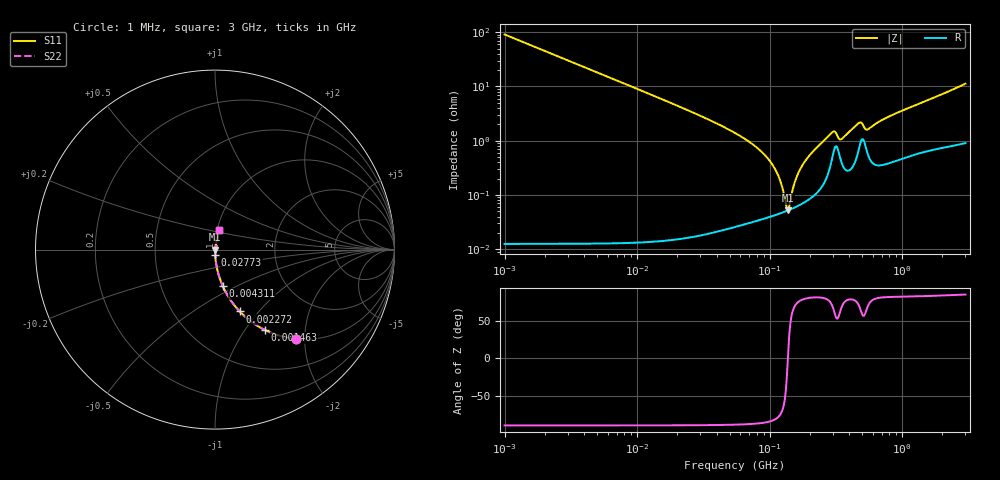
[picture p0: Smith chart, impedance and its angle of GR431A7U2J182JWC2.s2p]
!Murata Part Number: GR431A7U2J182JWC2
!These Parameters are Measured in Series Mode Connection
!Data Generated on Jun 10, 2025
!  o--ll--o
!Port1  Port2
!  o------o
!Operation Temp=25[degC], DC Bias Voltage=0[V]
!Freq. Start=1000[kHz] Stop=3[GHz] 401[Steps]
# Hz S RI R 50
!Freq.(Hz) S11(Real) S11(Imag) S21(Real) S21(Imag) S12(Real) S12(Imag) S22(Real) S22(Imag)
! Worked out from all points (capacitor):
!   401 points, 1 MHz to 3 GHz, reference 50 ohm
!   read as one part in series: C = 1.75 nF near 1.041 MHz
!   lowest |Z| = 52.1 mohm at 137.5 MHz (marker M1)
!   series resonance near 137.3 MHz, so ESL is about 770 pH
!   S11 on the Smith chart (normalised r, x): 1 MHz: 1.00, -1.82; 1.463 MHz: 1.00, -1.24; 2.272 MHz: 1.00, -0.80; 4.311 MHz: 1.00, -0.42; 27.73 MHz: 1.00, -0.06; 3 GHz: 1.02, +0.22
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1000000  0.4524 -0.4977  0.5476 0.4977  0.5476 0.4977  0.4524 -0.4977
1462727  0.2786 -0.4482  0.7214 0.4482  0.7214 0.4482  0.2786 -0.4482
2271982  0.138 -0.3447  0.862 0.3447  0.862 0.3447  0.138 -0.3447
3823119  0.0535 -0.2248  0.9465 0.2248  0.9465 0.2248  0.0535 -0.2248
4310966  0.0426 -0.2016  0.9574 0.2016  0.9574 0.2016  0.0426 -0.2016
1.461624e7  0.0039 -0.0612  0.9961 0.0612  0.9961 0.0612  0.0039 -0.0612
2.773354e7  0.00116 -0.0313  0.9988 0.0313  0.9988 0.0313  0.00116 -0.0313
5.477226e7  0.00045 -0.0139  0.9996 0.0139  0.9996 0.0139  0.00045 -0.0139
8.011685e7  0.000389 -0.00746  0.9996 0.00746  0.9996 0.00746  0.000389 -0.00746
1.018679e8  0.000415 -0.00401  0.9996 0.00401  0.9996 0.00401  0.000415 -0.00401
1.171891e8  0.000452 -0.00211  0.9995 0.00211  0.9995 0.00211  0.000452 -0.00211
1.321429e8  0.0005 -0.000506  0.9995 0.000506  0.9995 0.000506  0.0005 -0.000506
1.375402e8  0.00052 2.72e-05  0.9995 -2.72e-05  0.9995 -2.72e-05  0.00052 2.72e-05
1.403209e8  0.00053 0.000295  0.9995 -0.000295  0.9995 -0.000295  0.00053 0.000295
1.646891e8  0.00064 0.00247  0.9994 -0.00247  0.9994 -0.00247  0.00064 0.00247
2.094008e8  0.00095 0.00603  0.9991 -0.00603  0.9991 -0.00603  0.00095 0.00603
3.002264e8  0.00562 0.0134  0.9944 -0.0134  0.9944 -0.0134  0.00562 0.0134
3.453811e8  0.00435 0.00961  0.9957 -0.00961  0.9957 -0.00961  0.00435 0.00961
4.66327e8  0.00662 0.0196  0.9934 -0.0196  0.9934 -0.0196  0.00662 0.0196
5.473095e8  0.00606 0.0148  0.9939 -0.0148  0.9939 -0.0148  0.00606 0.0148
8.005644e8  0.00462 0.0277  0.9954 -0.0277  0.9954 -0.0277  0.00462 0.0277
3e9  0.021 0.1088  0.979 -0.1088  0.979 -0.1088  0.021 0.1088
